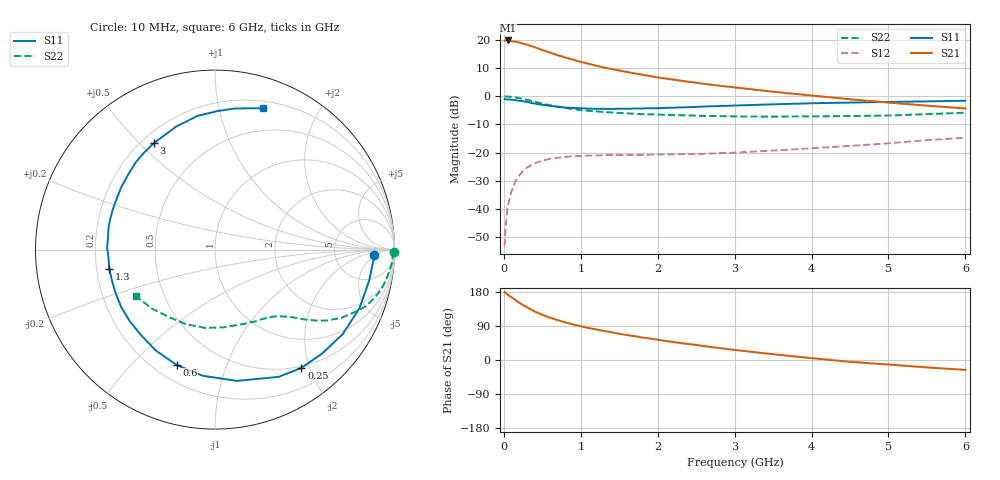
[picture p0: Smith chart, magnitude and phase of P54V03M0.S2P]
! SIEMENS Small Signal Semiconductors
! BFP183
! Si NPN RF Bipolar Junction Transistor in SOT143
! VCE = 4 V  IC = 3 mA
! Common Emitter S-Parameters:  March  1996
# GHz  S  MA  R  50
!  f  S11  S21  S12  S22
! GHz  MAG  ANG  MAG  ANG  MAG  ANG  MAG  ANG
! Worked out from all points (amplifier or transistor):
!   36 points, 10 MHz to 6 GHz, reference 50 ohm
!   highest |S21| = 19.8 dB at 50 MHz (marker M1)
!   |S21| within 3 dB of that: start of sweep to 460.4 MHz
!   unconditionally stable (mu >= 1): 1.885 GHz to 5.715 GHz
!   at 250 MHz: K = 0.15, MSG = 22.6 dB, |S12| = -26.5 dB
!   at 1.4 GHz: K = 0.78, MSG = 15.2 dB, |S12| = -20.9 dB
!   at 6 GHz: K = 0.94, MSG = 5.2 dB, |S12| = -14.7 dB
!   lowest NFmin = 1.10 dB at 450 MHz
!   S11 on the Smith chart (normalised r, x): 10 MHz: 15, -5; 250 MHz: 0.47, -1.87; 600 MHz: 0.29, -0.68; 1.3 GHz: 0.25, -0.08; 3 GHz: 0.25, +0.55; 6 GHz: 0.27, +1.37
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0.01  0.8887 -2.1  9.652 178.7  0.0022 88.4  0.9975 -0.9
0.02  0.8834 -4.6  9.738 177.5  0.0044 89.7  0.9911 -1.8
0.05  0.876 -11.4  9.753 172.5  0.011 84.4  0.9887 -4.5
0.15  0.8532 -33.6  9.293 158.0  0.0309 71.1  0.9543 -13.2
0.2  0.8315 -44.1  8.998 151.2  0.0394 66.6  0.9275 -17.0
0.25  0.8163 -53.9  8.535 144.9  0.0471 61.3  0.8986 -20.5
0.3  0.7925 -63.5  8.219 139.4  0.0542 56.9  0.8636 -23.3
0.4  0.7413 -80.6  7.427 128.1  0.0648 48.8  0.7995 -28.4
0.5  0.7059 -95.7  6.582 119.2  0.0721 42.2  0.7405 -32.2
0.6  0.6773 -108.4  5.958 111.8  0.0781 37.5  0.6936 -34.8
0.7  0.6518 -120.5  5.332 105.1  0.0813 33.8  0.6528 -36.9
0.8  0.6301 -130.7  4.885 99.2  0.0842 30.4  0.6204 -38.6
0.9  0.6204 -139.9  4.462 94.0  0.0862 27.9  0.5913 -40.0
1.1  0.6047 -156.2  3.766 84.5  0.0886 24.0  0.5514 -42.6
1.3  0.5986 -169.7  3.239 76.8  0.0902 21.4  0.5266 -44.9
1.6  0.6002 173.3  2.696 65.9  0.091 19.6  0.4981 -48.5
2.2  0.6274 146.4  1.974 47.4  0.0931 19.8  0.4635 -57.5
3  0.6841 119.9  1.435 26.6  0.1001 23.0  0.4387 -72.8
3.5  0.7188 107.5  1.205 15.2  0.1089 25.0  0.4357 -83.8
4.5  0.7723 88.9  0.885 -4.8  0.1319 25.6  0.4458 -110.9
5.5  0.8105 76.3  0.682 -19.6  0.1669 23.2  0.4822 -137.2
6  0.8323 71.1  0.607 -26.1  0.1836 19.5  0.5104 -149.5
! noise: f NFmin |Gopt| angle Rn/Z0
0.45  1.1  0.37  35  0.3
0.9  1.15  0.34  85  0.23
1.8  1.9  0.35  160  0.13
